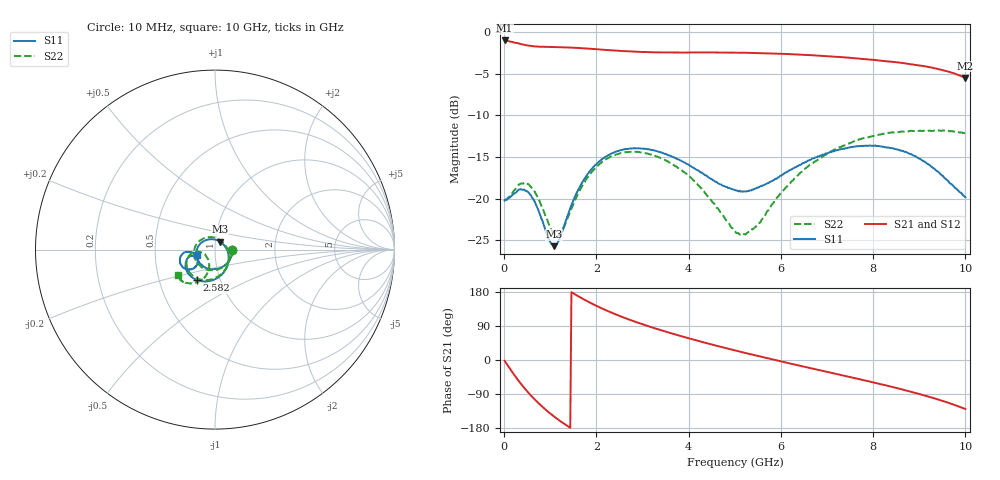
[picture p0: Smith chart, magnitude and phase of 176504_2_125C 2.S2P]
!  2-Port S-parameters saved by WinCal
! VAR MeasName=S-Parameters (CALIBRATED_DATA) read from VNA (N5242A)
! VAR MeasDate=2017-11-2 17:34:48
! VAR NAME=176504_2_125C 2
! VAR FILENAME=176504_2_125C 2.S2P
! VAR DATE=2017-11-2 17:34:48
! VAR PHYS_PORTS=2,3
# Hz S DB R 50
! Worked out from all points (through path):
!   401 points, 10 MHz to 10 GHz, reference 50 ohm
!   highest |S21| = -1.02 dB at 10 MHz (marker M1); lowest = -5.5 dB at 10 GHz (marker M2)
!   lowest |S11| = -25.7 dB at 1.084 GHz (marker M3), VSWR 1.11, Z = 52.6 + j4.65 ohm
!   |S11| at or under -10 dB: start of sweep to end of sweep
!   |S22| runs from -24.5 to -11.8 dB; largest |S21 - S12| = 0.013
!   S11 on the Smith chart (normalised r, x): 10 MHz: 1.22, -0.01; 2.582 GHz: 0.77, -0.27; 10 GHz: 0.82, -0.05
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1e7  -20.21 -2.5  -1.02 -2.2  -1.02 -2.2  -20.22 -2.4
1.34875e8  -19.82 -52.3  -1.15 -24.7  -1.15 -24.7  -19.67 -55.0
2.5975e8  -19.25 -93.6  -1.32 -46.1  -1.32 -46.1  -18.76 -96.8
4.5955e8  -19.05 -145.3  -1.57 -77.0  -1.57 -77.0  -18.20 -148.3
7.34275e8  -21.27 155.4  -1.76 -112.6  -1.76 -112.6  -19.91 154.1
9.091e8  -23.96 113.8  -1.79 -132.0  -1.79 -131.9  -22.24 116.3
1.083925e9  -25.69 58.1  -1.81 -149.3  -1.80 -149.2  -24.31 67.9
1.2088e9  -24.68 18.6  -1.82 -160.6  -1.82 -160.5  -24.25 29.9
1.35865e9  -22.31 -16.2  -1.85 -173.1  -1.85 -173.1  -22.60 -8.1
1.683325e9  -18.15 -60.4  -1.95 162.9  -1.95 163.0  -18.57 -57.8
2.1079e9  -15.32 -94.7  -2.12 136.8  -2.11 136.8  -15.67 -94.7
2.582425e9  -14.11 -120.8  -2.29 112.5  -2.29 112.7  -14.49 -122.6
3.35665e9  -14.38 -148.7  -2.45 80.3  -2.47 80.5  -15.03 -153.5
4.230775e9  -16.71 -164.7  -2.45 49.6  -2.45 50.1  -18.50 -173.1
5.005e9  -18.98 -158.1  -2.47 25.3  -2.47 25.6  -23.88 -157.4
5.379625e9  -18.90 -148.1  -2.51 14.1  -2.51 14.5  -23.63 -128.8
6.05395e9  -17.06 -138.7  -2.63 -5.2  -2.64 -4.7  -18.99 -107.0
6.678325e9  -15.19 -140.7  -2.79 -22.4  -2.81 -22.1  -15.73 -110.0
7.577425e9  -13.77 -151.3  -3.15 -47.2  -3.17 -46.9  -13.12 -122.4
8.35165e9  -13.91 -164.8  -3.54 -69.2  -3.60 -68.7  -12.11 -132.2
9.2008e9  -15.88 -175.4  -4.19 -96.6  -4.22 -95.7  -11.85 -139.7
1e10  -19.82 -164.3  -5.53 -129.3  -5.54 -128.4  -12.16 -145.6
